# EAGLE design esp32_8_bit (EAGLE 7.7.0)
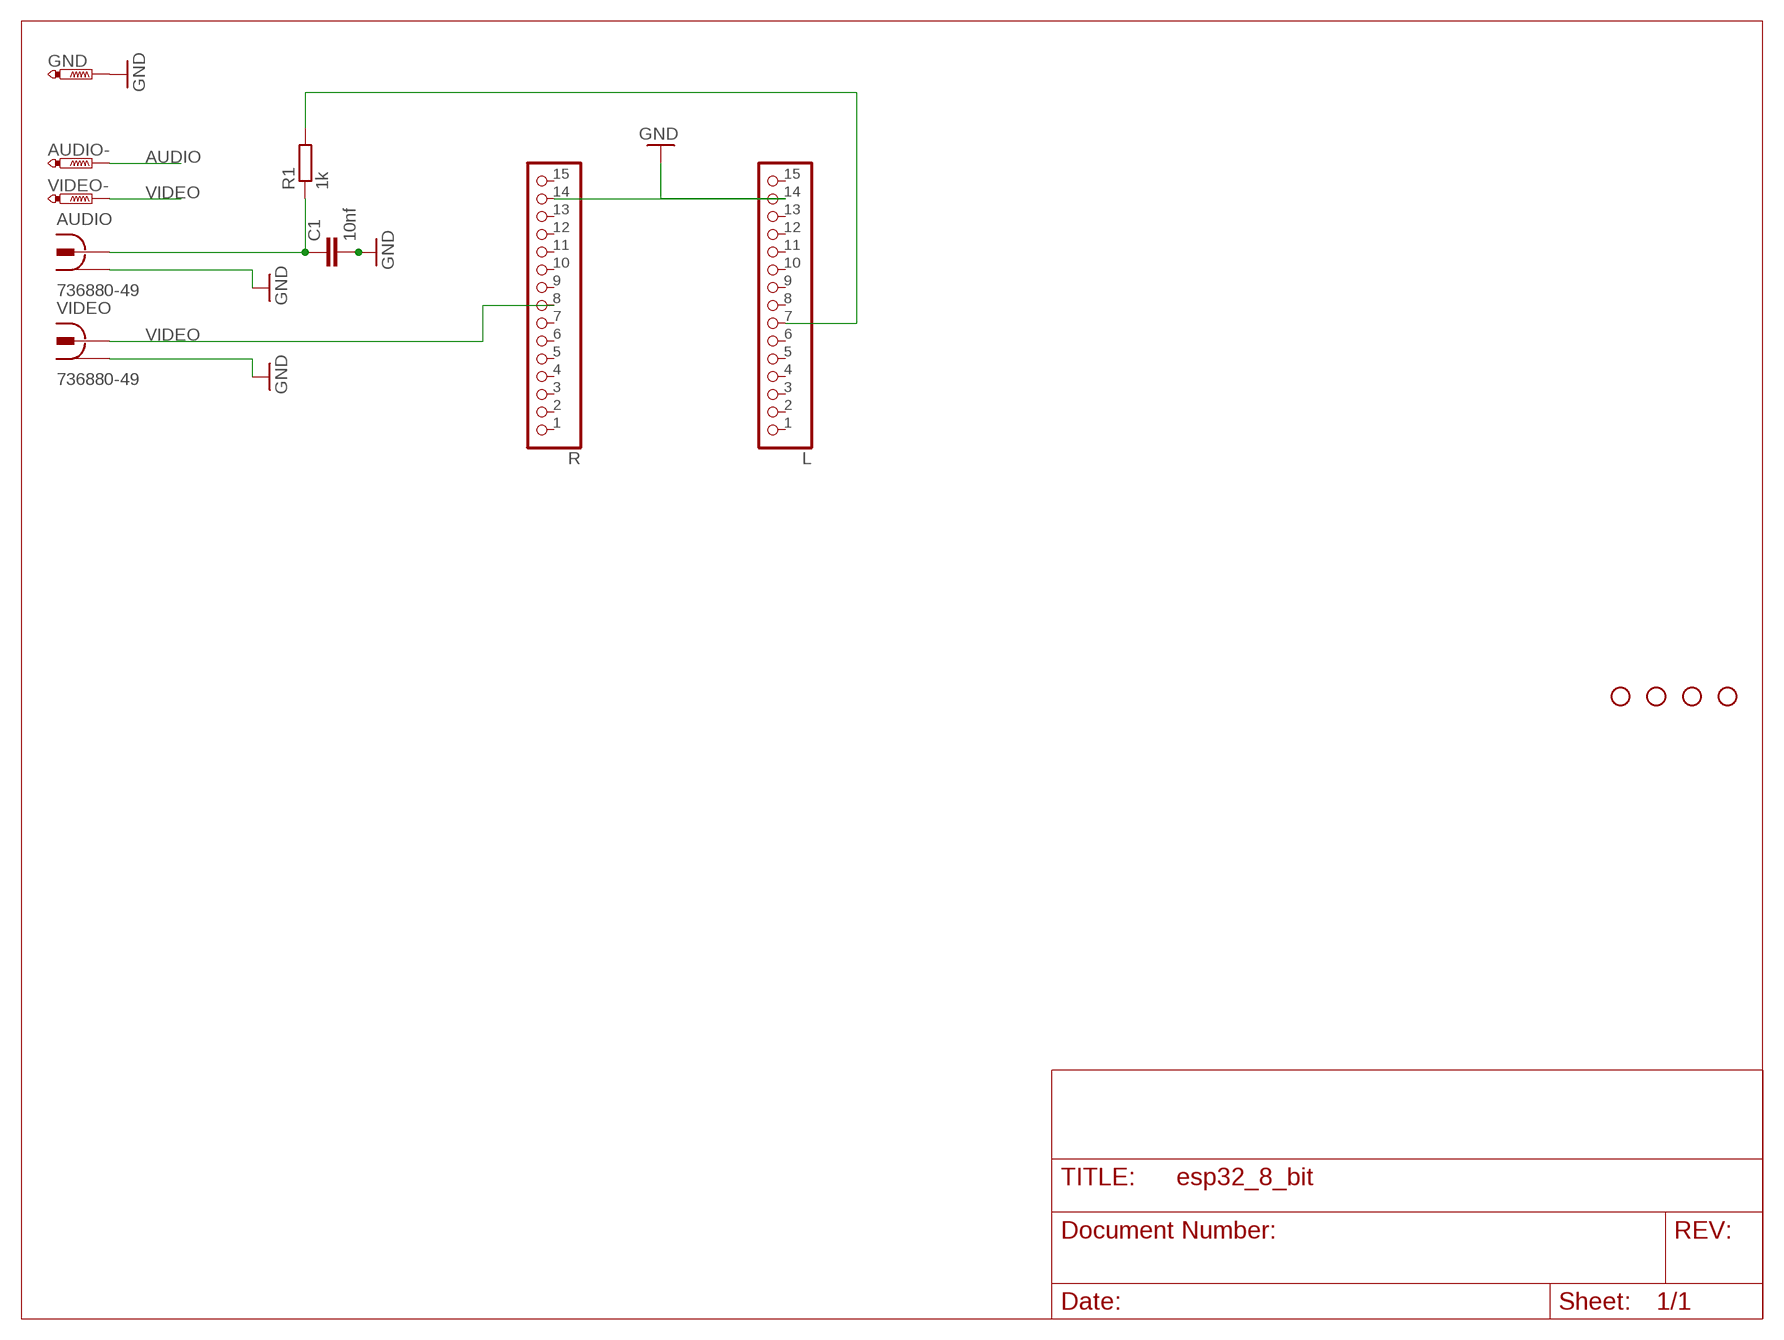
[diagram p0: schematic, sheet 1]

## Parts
AUDIO  736880-49  [736880-49]
AUDIO-  PTR1PAD1-20Y  [P1-20Y]
C1  10nf  C-EU050-024X044  [C050-024X044]
GND  PTR1PAD1-20Y  [P1-20Y]
L  PINHD-1X15  [1X15]
R  PINHD-1X15  [1X15]
R1  1k  R-EU_0207/10  [0207/10]
U$2  STAND-OFF  [STAND-OFF]
U$3  STAND-OFF  [STAND-OFF]
U$4  STAND-OFF  [STAND-OFF]
U$5  STAND-OFF  [STAND-OFF]
VIDEO  736880-49  [736880-49]
VIDEO-  PTR1PAD1-20Y  [P1-20Y]

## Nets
AUDIO: AUDIO-.1(TP) AUDIO.2 C1.1 R1.1
GND: AUDIO.1 AUDIO.1@1 AUDIO.1@2 C1.2 GND.1(TP) L.14 R.14 VIDEO.1 VIDEO.1@1 VIDEO.1@2
N$1: L.7 R1.2
VIDEO: R.8 VIDEO-.1(TP) VIDEO.2
Unconnected: L.1 L.2 L.3 L.4 L.5 L.6 L.8 L.9 L.10 L.11 L.12 L.13 L.15 R.1 R.2 R.3 R.4 R.5 R.6 R.7 R.9 R.10 R.11 R.12 R.13 R.15

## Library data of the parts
AUDIO VIDEO = con-conrad:736880-49: Cinch Connector ( RCA Jack )
AUDIO- GND VIDEO- = testpad:PTR1: TEST PIN
C1 = rcl:C-EU: CAPACITOR, European symbol
L R = pinhead:PINHD-1X15: PIN HEADER
R1 = resistor:R-EU_: RESISTOR, European symbol
U$2-U$5 = SparkFun:STAND-OFF: Stand Off

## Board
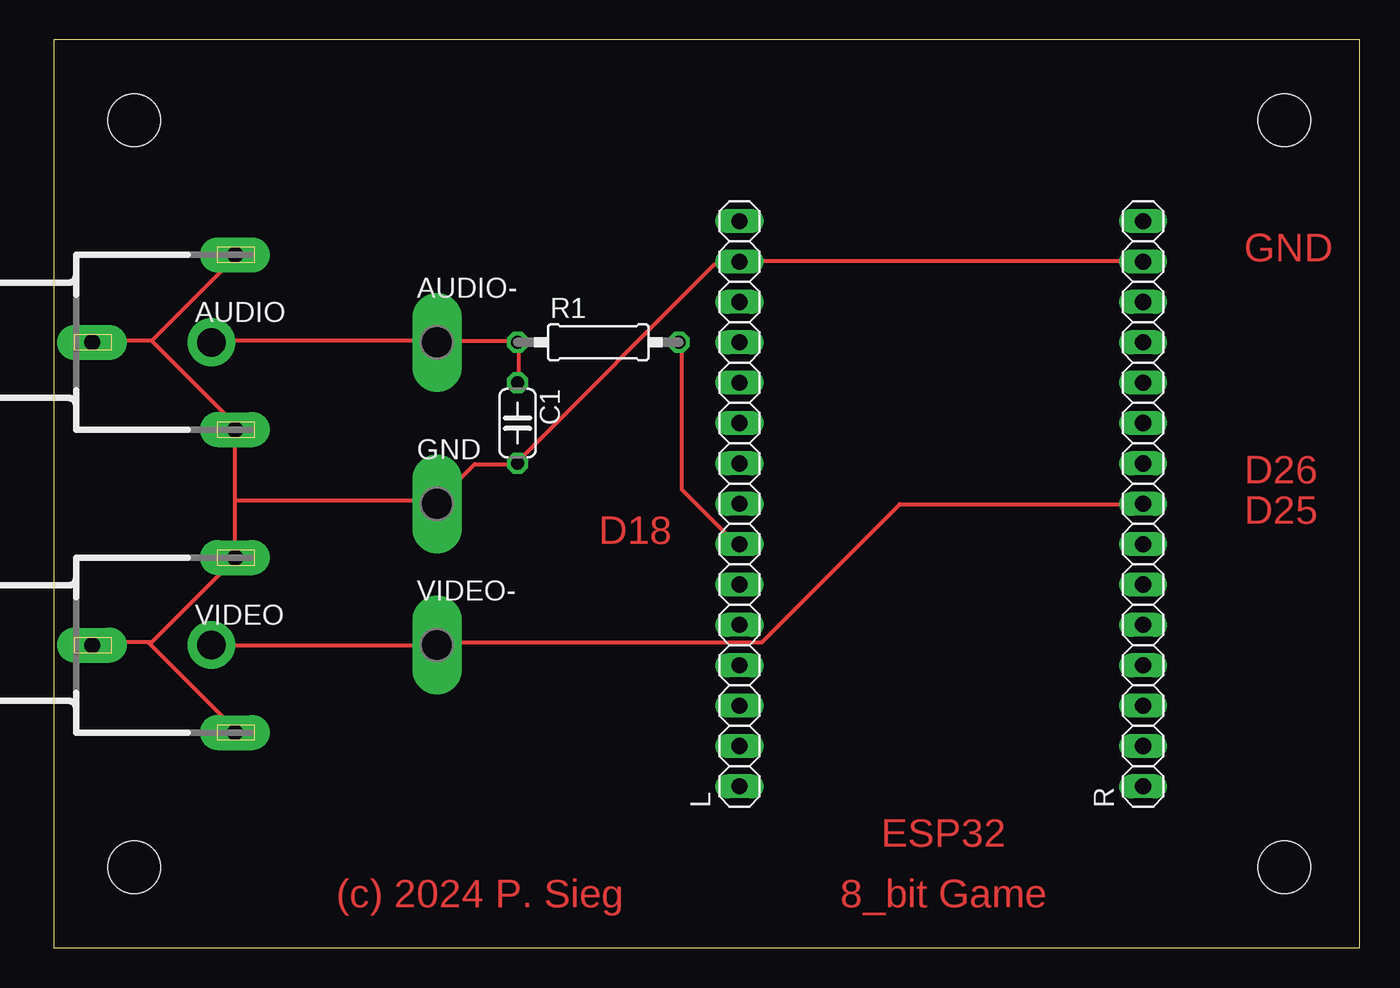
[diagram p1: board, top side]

Size 82.22 x 57.14 mm. Coordinates in mm from the lower left corner, seen from the top.
Outline: 0,0 82.22,0 82.22,57.14 0,57.14 0,0
Copper layers (1*16): Top 0.035mm / dielectric 1.5mm / Bottom 0.035mm
Design rules "default": minimum track width 10mil, minimum drill 24mil, track to track 8mil, track to pad 8mil, pad to pad 8mil, via to via 8mil, smd to smd 8mil, copper to edge 40mil, drill to drill 8mil, minimum pad ring 10mil, minimum via ring 8mil, stop-mask expansion 4mil, vias tented up to drill 0mil, thermal gap 10mil

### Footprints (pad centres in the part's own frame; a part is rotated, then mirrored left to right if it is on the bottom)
736880-49 = drill 1 pad 2.2 long: 1 -3.92,0; 1@1 5.08,-5.5; 1@2 5.08,5.5 | drill 1.8 pad 3: 2 3.58,0
P1-20Y = drill 2.1 pad 2.54 long: 1 0,0
C050-024X044 = drill 0.813 octagon: 1 -2.54,0; 2 2.54,0
1X15 = drill 1.016 long: 1 -17.78,0; 2 -15.24,0; 3 -12.7,0; 4 -10.16,0; 5 -7.62,0; 6 -5.08,0; 7 -2.54,0; 8 0,0; 9 2.54,0; 10 5.08,0; 11 7.62,0; 12 10.16,0; 13 12.7,0; 14 15.24,0; 15 17.78,0
0207/10 = drill 0.813 octagon: 1 -5.08,0; 2 5.08,0
STAND-OFF = hole 3.302: 0,0

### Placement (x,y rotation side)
AUDIO  6.35,38.1 0 top
AUDIO-  24.13,38.1 0 top
C1  29.21,33.02 270 top
GND  24.13,27.94 0 top
L  43.18,27.94 90 top
R  68.58,27.94 90 top
R1  34.29,38.1 0 top
U$2  77.47,5.08 0 top
U$3  5.08,5.08 0 top
U$4  77.47,52.07 0 top
U$5  5.08,52.07 0 top
VIDEO  6.35,19.05 0 top
VIDEO-  24.13,19.05 0 top

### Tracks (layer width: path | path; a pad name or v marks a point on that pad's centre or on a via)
AUDIO
  Top 0.254: C1.1 29.26,35.69 29.26,37.97 R1.1 29.03,38.2 24.23,38.2 AUDIO-.1 24,38.2 10.06,38.2 AUDIO.2
GND
  Top 0.254: 6.17,38.2 2.52,38.2 AUDIO.1 | 6.17,38.2 11.43,43.46 AUDIO.1@2 | 5.94,19.23 6.17,19.23 11.43,24.49 VIDEO.1@2 11.43,28.14 | 5.94,19.23 2.52,19.23 VIDEO.1 | 5.94,19.23 11.43,13.74 VIDEO.1@1 | 11.43,28.14 AUDIO.1@1 11.43,32.94 6.17,38.2 | R.14 68.58,43.23 43.2,43.23 L.14 42.98,43 41.6,43 29.26,30.66 C1.2 29.03,30.43 26.52,30.43 24.23,28.14 GND.1 24,28.14 11.43,28.14
N$1
  Top 0.254: R1.2 39.55,37.97 39.55,28.83 42.98,25.4 L.7
VIDEO
  Top 0.254: R.8 68.58,27.91 53.26,27.91 44.58,19.23 24.23,19.23 VIDEO-.1 24,19 10.06,19 VIDEO.2

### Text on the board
Top: GND | D26 | D25 | D18 | ESP32 | (c) 2024 P. Sieg | 8_bit Game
